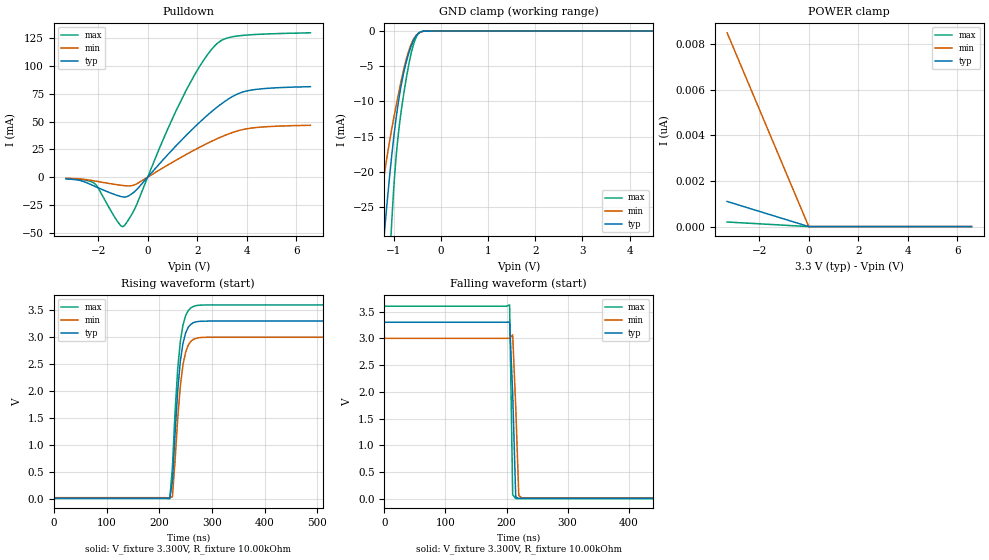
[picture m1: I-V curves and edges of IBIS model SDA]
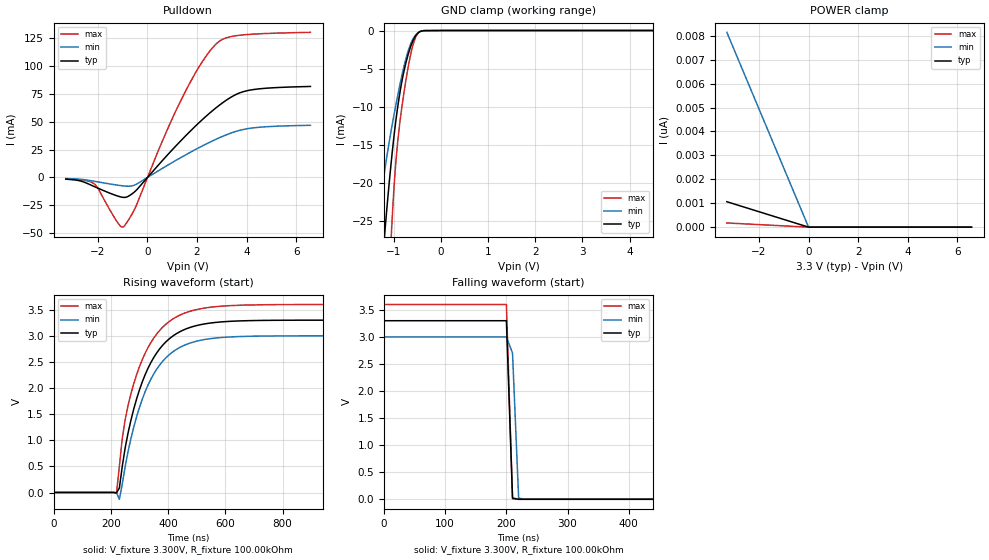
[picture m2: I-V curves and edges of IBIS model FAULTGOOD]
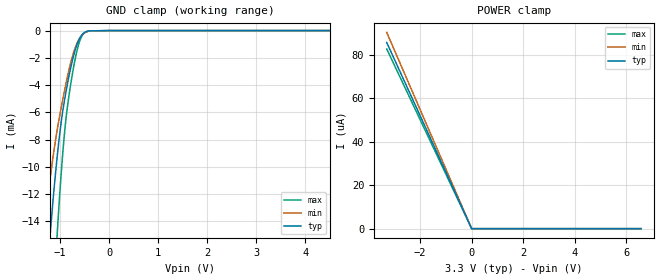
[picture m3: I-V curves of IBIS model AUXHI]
|Texas Instruments Incorporated
|PCIExpress Server Dual Slot Hot Plug Controller
| Marketing part#   Voltage Range   Package-type   Temperature
|TPS2363PFBR   AUXINA/B(3.0V-3.6V)  48-pin TQFP   -40C to 125C(Junction)
[IBIS Ver]   4.0
[File name]   tps2363.ibs
[File Rev]   1.0
[Date]   03/10/2009
[Source]   Texas Instruments Incorporated.
   Analog-eLab, HPA
   12500 TI Blvd
   Dallas, TX -75243
   For Support e-mail: elab_ibis@list.ti.com
[Notes]   Revision History:
   1.0: 03/10/2009
   - Model based on Simulations in TISPICE
   - C_comp for typ, min, max for all models are based on
   PVT corner conditions, warnings can be ignored
   - Warnings related to Ax's POWERCLAMP data reflects true
   buffer behavior, hence can be ignored
   - Model not matched to measurements
[Disclaimer]
 This product is designed as an aid for customers of Texas Instruments.
 No warranties, either expressed or implied, with respect to this third
 party software (if any) or with respect to its fitness for any
 particular purpose is claimed by Texas Instruments or the author. The
 software (if any) is provided solely on an "as is" basis. The entire
 risk as to its quality and performance is with the customer
[Copyright] (C) Copyright 2009 Texas Instruments Incorporated.
   All rights reserved.
|   TPS2363PFB 48-pin TQFP
[Component]   TPS2363PFB
[Manufacturer]  Texas Instruments Incorporated
[Package]   |48-pin TQFP
|   typ   min   max
R_pkg   59.77m   54.34m   65.19m
L_pkg   3.606nH   3.263nH   3.950nH
C_pkg   0.558pF   0.522pF   0.595pF
[Pin]   signal_name   model_name   R_pin   L_pin   C_pin
   1   FAULTA_   FAULTGOOD   0.06008   3.79042nH   0.54184pF
   2   FILTERA_   NC   0.05750   3.57782nH   0.57905pF
   3   G12A   NC   0.05750   3.51101nH   0.55666pF
   4   GPIA1   GPI   0.05527   3.37783nH   0.53806pF
   5   SH12A   NC   0.05659   3.51920nH   0.57502pF
   6   PGOODA_   FAULTGOOD   0.05514   3.30066nH   0.52228pF
   7   GPIA2   GPI   0.05567   3.31899nH   0.52322pF
   8   SL12A   NC   0.05806   3.56898nH   0.57967pF
   9   FORCEONA_   NC   0.05776   3.46263nH   0.54642pF
   10   OUT12A   NC   0.06086   3.62608nH   0.57132pF
   11   AUXINA   POWER   0.03321   3.44900nH   0.63242pF
   12   SH33A   NC   0.06177   3.85072nH   0.54570pF
   13   SL33A   NC   0.06072   3.81350nH   0.54385pF
   14   G33A   NC   0.05536   3.50872nH   0.57094pF
   15   VUXA   NC   0.03651   3.71715nH   0.60146pF
   16   OUT33A   NC   0.05464   3.35756nH   0.53113pF
   17   GND   GND   0.05434   3.44537nH   0.57047pF
   18   AUXHIA   AUXHI   0.05436   3.27585nH   0.52197pF
   19   AUXHIB   AUXHI   0.05484   3.29122nH   0.52319pF
   20   RFILTERAB   NC   0.05589   3.49637nH   0.57461pF
   21   OUT33B   NC   0.05693   3.43257nH   0.53380pF
   22   VAUXB   NC   0.03653   3.71803nH   0.59673pF
   23   G33B   NC   0.05543   3.51198nH   0.57137pF
   24   SL33B   NC   0.06074   3.81536nH   0.54409pF
   25   SH33B   NC   0.06175   3.84570nH   0.54605pF
   26   AUXINB   POWER   0.03316   3.44261nH   0.63209pF
   27   OUT12B   NC   0.06089   3.62061nH   0.57134pF
   28   FORCEONB_   NC   0.05780   3.45785nH   0.54718pF
   29   SL12B   NC   0.05807   3.56322nH   0.58092pF
   30   GPIB2   GPI   0.05565   3.31265nH   0.52431pF
   31   PGOODB_   NC   0.05512   3.29432nH   0.52293pF
   32   SH12B   NC   0.05659   3.51277nH   0.57506pF
   33   GND   GND   0.05542   3.37577nH   0.53853pF
   34   G12B   NC   0.05737   3.50025nH   0.55829pF
   35   FILTERB   NC   0.05750   3.57098nH   0.58170pF
   36   FAULTB_   FAULTGOOD   0.06022   3.78876nH   0.54193pF
   37   INT_   NC   0.06519   3.95031nH   0.55519pF
   38   GPIB1   GPI   0.06153   3.70017nH   0.59485pF
   39   A2   Ax   0.05889   3.54586nH   0.56592pF
   40   A1   Ax   0.05697   3.42176nH   0.54600pF
   41   A0   Ax   0.05588   3.48296nH   0.57533pF
   42   AUXENB   INPUT   0.05481   3.27747nH   0.52308pF
   43   ONB   INPUT   0.05434   3.26250nH   0.52163pF
   44   ONA   INPUT   0.05449   3.43779nH   0.57079pF
   45   AUXENA   INPUT   0.05468   3.34695nH   0.53878pF
   46   GND   GND   0.05620   3.45768nH   0.55715pF
   47   SCL   INPUT   0.05765   3.57325nH   0.58249pF
   48   SDA   SDA   0.06059   3.79947nH   0.54479pF
| Models and submodels in the file (6): SDA (I/O_open_drain), FAULTGOOD (Open_drain), AUXHI (Input), Ax (Input), GPI (Input), INPUT (Input)
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|   SDA MODEL
[Model]   SDA
Model_type   I/O_open_drain
Vinl = 0.8V
Vinh = 2.0V
Vmeas = 3.3V
Vref = 3.3V
Cref = 0.000pF
Rref = 0.0Ohm
C_comp   3.397pF   3.518pF   3.290pF
[Voltage Range]   3.300V   3.000V   3.600V
|Junction Temperature
[Temperature Range]   40.0   125.0   -40.0
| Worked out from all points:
|   slope of the pulldown table from 0 to 0.495 V, typ, clamps not added: 39.7 ohm
|   GND clamp passes 1 mA (typ) near -0.56 V on its own axis
|   falling waveform, V_fixture 3.300V, R_fixture 10.00kOhm: 20-80 % time 5.88ns typ, 5.88ns min, 3.04ns max; typ from 3.3 V to 0.013 V
|   rising waveform, V_fixture 3.300V, R_fixture 10.00kOhm: 20-80 % time 14.3ns typ, 14.6ns min, 13.9ns max; typ from 0.013 V to 3.3 V
[Pulldown]
|   Voltage   I(typ)   I(min)   I(max)
-3.3V     -1.487mA   -948uA     -1.347mA
-2.142V   -8.198mA   -3.42mA    -5.758mA
-1.231V   -16.44mA   -6.825mA   -39.55mA
-953.7mV  -17.87mA   -7.608mA   -43.87mA
-488.4mV  -12.19mA   -6.485mA   -26.89mA
580.8mV   14.6mA     7.86mA     31.53mA
1.551V    37.52mA    20.34mA    77.96mA
2.076V    48.9mA     26.64mA    98.78mA
2.689V    60.93mA    33.4mA     117.7mA
3.165V    68.88mA    38mA       124.9mA
3.977V    77.43mA    43.42mA    127.9mA
6.58V     81.47mA    46.7mA     129.9mA
[GND Clamp]
|   Voltage   I(typ)   I(min)   I(max)
-3.3V     -270.2mA   -171.7mA   -480.3mA
-1.36V    -41.93mA   -28.02mA   -76.34mA
-1.191V   -28.08mA   -19.96mA   -48.24mA
-1.053V   -18.29mA   -14.27mA   -28.3mA
-993.3mV  -14.69mA   -12.1mA    -21.59mA
-943.8mV  -12.05mA   -10.37mA   -17.35mA
-874.5mV  -8.933mA   -8.059mA   -12.98mA
-805.2mV  -6.416mA   -5.912mA   -9.646mA
-617.1mV  -1.868mA   -1.624mA   -2.751mA
-518.1mV  -610.3uA   -546.3uA   -772.6uA
-419.1mV  -98.09uA   -114.5uA   -74.94uA
6.58V     0A         0A         0A
[POWER Clamp]
|   Voltage   I(typ)   I(min)   I(max)
-3.3V     1.101nA    8.484nA    200.7pA
0V        0A         0A         0A
6.58V     0A         0A         0A
[Ramp]
R_load = 10.00kOhm
|   typ   min   max
dV/dt_r   1.972V/14.331ns   1.787V/14.621ns   2.156V/13.926ns
dV/dt_f   1.972V/5.880ns   1.787V/5.875ns   2.156V/3.043ns
[Falling Waveform]
V_fixture = 3.300V
V_fixture_min = 3.000V
V_fixture_max = 3.600V
R_fixture = 10.00kOhm
|   Time   V(typ)   V(min)   V(max)
0s        3.3V       3V         3.6V
200ns     3.3V       3V         3.6V
205ns     3.305V     3V         3.624V
210ns     1.972V     3.063V     80.67mV
215ns     36.77mV    1.723V     6.733mV
220ns     12.35mV    64.2mV     7.022mV
225ns     13.49mV    21.94mV    6.363mV
1.25us    12.85mV    21.69mV    6.387mV
[Rising Waveform]
V_fixture = 3.300V
V_fixture_min = 3.000V
V_fixture_max = 3.600V
R_fixture = 10.00kOhm
|   Time   V(typ)   V(min)   V(max)
0s        12.85mV    21.69mV    6.387mV
220ns     10.72mV    20.65mV    3.217mV
225ns     319.7mV    39.33mV    586.5mV
230ns     1.206V     708.4mV    1.61V
235ns     2.006V     1.49V      2.409V
240ns     2.555V     2.094V     2.922V
245ns     2.889V     2.488V     3.227V
250ns     3.08V      2.722V     3.4V
265ns     3.272V     2.962V     3.574V
1.25us    3.3V       3V         3.6V
|   FAULTGOOD MODEL
[Model]   FAULTGOOD
Model_type   Open_drain
Vmeas = 3.3V
Vref = 3.3V
Cref = 0.000pF
Rref = 0.0Ohm
C_comp   3.256pF   3.378pF   3.147pF
[Voltage Range]   3.300V   3.000V   3.600V
|Junction Temperature
[Temperature Range]   40.0   125.0   -40.0
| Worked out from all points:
|   slope of the pulldown table from 0 to 0.495 V, typ, clamps not added: 39.7 ohm
|   GND clamp passes 1 mA (typ) near -0.56 V on its own axis
|   falling waveform, V_fixture 3.300V, R_fixture 100.00kOhm: 20-80 % time 6.04ns typ, 6.71ns min, 6.01ns max; typ from 3.3 V to 0.001 V
|   rising waveform, V_fixture 3.300V, R_fixture 100.00kOhm: 20-80 % time 112ns typ, 111ns min, 107ns max; typ from 0.001 V to 3.3 V
[Pulldown]
|   Voltage   I(typ)   I(min)   I(max)
-3.3V     -1.487mA   -948uA     -1.347mA
-2.142V   -8.198mA   -3.42mA    -5.758mA
-1.231V   -16.44mA   -6.825mA   -39.55mA
-953.7mV  -17.87mA   -7.608mA   -43.87mA
-488.4mV  -12.19mA   -6.485mA   -26.89mA
580.8mV   14.6mA     7.86mA     31.53mA
1.551V    37.52mA    20.34mA    77.96mA
2.076V    48.9mA     26.64mA    98.78mA
2.689V    60.93mA    33.4mA     117.7mA
3.165V    68.88mA    38mA       124.9mA
3.977V    77.43mA    43.42mA    127.9mA
6.58V     81.47mA    46.7mA     129.9mA
[GND Clamp]
|   Voltage   I(typ)   I(min)   I(max)
-3.3V     -264mA     -165.2mA   -473.8mA
-1.369V   -41.32mA   -26.75mA   -76.74mA
-1.35V    -39.64mA   -25.79mA   -73.32mA
-1.201V   -27.76mA   -19.02mA   -48.85mA
-1.162V   -24.85mA   -17.37mA   -42.77mA
-1.043V   -16.93mA   -12.88mA   -26.39mA
-983.4mV  -13.53mA   -10.87mA   -20.04mA
-924mV    -10.61mA   -8.949mA   -15.43mA
-775.5mV  -5.253mA   -4.63mA    -8.032mA
-587.4mV  -1.326mA   -1.102mA   -1.894mA
-419.1mV  -91.93uA   -105.7uA   -67.18uA
6.58V     0A         0A         0A
[POWER Clamp]
|   Voltage   I(typ)   I(min)   I(max)
-3.3V     1.064nA    8.146nA    175.5pA
0V        0A         0A         0A
6.58V     0A         0A         0A
[Ramp]
R_load = 100.00kOhm
|   typ   min   max
dV/dt_r   1.981V/111.818ns   1.800V/111.486ns   2.161V/106.878ns
dV/dt_f   1.981V/6.044ns   1.800V/6.715ns   2.161V/6.014ns
[Falling Waveform]
V_fixture = 3.300V
V_fixture_min = 3.000V
V_fixture_max = 3.600V
R_fixture = 100.00kOhm
|   Time   V(typ)   V(min)   V(max)
0s        3.303V     3.003V     3.603V
200ns     3.303V     3.003V     3.603V
210ns     25.03mV    2.704V     9.199mV
220ns     1.216mV    22.76mV    210.5uV
230ns     1.348mV    1.251mV    474.9uV
1.25us    1.288mV    2.181mV    639.9uV
[Rising Waveform]
V_fixture = 3.300V
V_fixture_min = 3.000V
V_fixture_max = 3.600V
R_fixture = 100.00kOhm
|   Time   V(typ)   V(min)   V(max)
0s        1.288mV    2.181mV    639.9uV
220ns     -5.901mV   -2.678mV   -13.33mV
230ns     88.24mV    -130.4mV   503.8mV
240ns     497.9mV    158.3mV    1.032V
250ns     848.9mV    488.8mV    1.391V
290ns     1.791V     1.449V     2.255V
350ns     2.587V     2.272V     2.959V
430ns     3.047V     2.745V     3.368V
610ns     3.278V     2.979V     3.579V
1.25us    3.303V     3.003V     3.603V
|   AUXHI MODEL
[Model]   AUXHI
Model_type   Input
Vinl = 0.8V
Vinh = 2.0V
|   typ   min   max
C_comp   2.678pF   2.813pF   2.553pF
[Voltage Range]   3.300V   3.000V   3.600V
|Junction Temperature
[Temperature Range]   40.0   125.0   -40.0
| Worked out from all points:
|   GND clamp passes 1 mA (typ) near -0.65 V on its own axis
[GND Clamp]
|   Voltage   I(typ)   I(min)   I(max)
-3.3V     -183.6mA   -124.9mA   -260mA
-1.34V    -21.72mA   -15.04mA   -35.42mA
-1.191V   -14.48mA   -10.53mA   -23.69mA
-1.063V   -9.367mA   -7.365mA   -15.13mA
-1.053V   -9.026mA   -7.153mA   -14.55mA
-983.4mV  -6.882mA   -5.765mA   -10.78mA
-924mV    -5.412mA   -4.663mA   -8.075mA
-815.1mV  -3.265mA   -2.828mA   -4.676mA
-716.1mV  -1.724mA   -1.515mA   -2.51mA
-617.1mV  -678uA     -651.6uA   -944.5uA
-468.6mV  -78.27uA   -103.7uA   -83.41uA
6.58V     0A         0A         0A
[POWER Clamp]
|   Voltage   I(typ)   I(min)   I(max)
-3.3V     85.57uA    90.2uA     82.59uA
-3.29V    85.28uA    89.89uA    82.3uA
0V        0A         0A         0A
6.58V     0A         0A         0A
